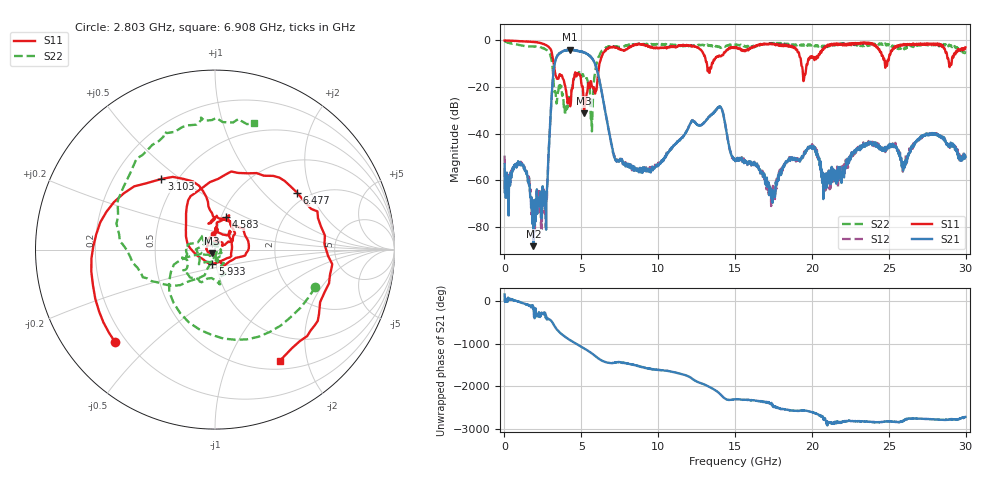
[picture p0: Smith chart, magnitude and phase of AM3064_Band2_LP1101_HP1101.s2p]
# Hz S DB R 50.0
!freq dBS11 angS11 dBS21 angS21 dBS12 angS12 dBS22 angS22
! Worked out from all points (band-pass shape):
!   1600 points, 10 MHz to 29.98 GHz, reference 50 ohm
!   highest |S21| = -4.03 dB at 4.246 GHz (marker M1); lowest = -88.3 dB at 1.884 GHz (marker M2)
!   |S21| within 3 dB of the highest: 3.401 GHz to 5.601 GHz (2.199 GHz wide, 48.9 % of centre)
!   lowest |S11| = -31.3 dB at 5.183 GHz (marker M3), VSWR 1.06, Z = 48.3 - j2.06 ohm
!   |S11| at or under -10 dB: 3.205 GHz to 6.181 GHz (2.975 GHz wide, 63.4 % of centre); 13.17 GHz to 13.49 GHz (325.6 MHz wide, 2.44 % of centre); 19.31 GHz to 19.71 GHz (406.2 MHz wide, 2.08 % of centre)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
!   |S22| runs from -39.1 to -0.3 dB; largest |S21 - S12| = 0.016
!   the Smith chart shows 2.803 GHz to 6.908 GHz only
!   S11 on the Smith chart (normalised r, x): 2.803 GHz: 0.16, -0.38; 3.103 GHz: 0.41, +0.43; 4.583 GHz: 1.06, +0.40; 5.933 GHz: 0.96, -0.15; 6.477 GHz: 1.75, +1.61; 6.908 GHz: 0.61, -1.56
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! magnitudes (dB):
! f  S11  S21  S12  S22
! 10 MHz  -0.1  -53.2  -49.5  -0.3
! 1.153 GHz  -0.4  -53.6  -53.5  -2.3
! 1.884 GHz  -0.7  -88.3  -72.9  -2.6
! 2.803 GHz  -2.4  -60.1  -59.1  -4.5
! 3.103 GHz  -6.1  -20.7  -20.7  -10.1
! 3.421 GHz  -16.5  -6.8  -6.9  -25.4
! 4.246 GHz  -26.5  -4.0  -4.1  -26.1
! 4.583 GHz  -14.4  -4.4  -4.4  -14.3
! 5.015 GHz  -18.8  -4.9  -4.8  -15.5
! 5.183 GHz  -31.3  -5.2  -5.1  -15.9
! 5.652 GHz  -18.4  -7.3  -7.3  -32.9
! 5.933 GHz  -21.9  -10.9  -10.9  -11.9
! 6.477 GHz  -5.1  -27.7  -27.6  -3.6
! 6.908 GHz  -2.9  -42.6  -42.4  -2.6
! 10 GHz  -3.4  -53.9  -53.7  -1.8
! 13.97 GHz  -6.5  -28.8  -28.5  -2.7
! 15 GHz  -3.0  -51.8  -51.4  -1.9
! 17.48 GHz  -1.5  -66.8  -63.2  -1.1
! 19.99 GHz  -6.8  -45.7  -45.5  -1.7
! 20.85 GHz  -3.1  -63.4  -61.8  -2.5
! 25 GHz  -8.2  -45.9  -45.6  -1.7
! 29.98 GHz  -3.0  -50.0  -50.5  -4.7
